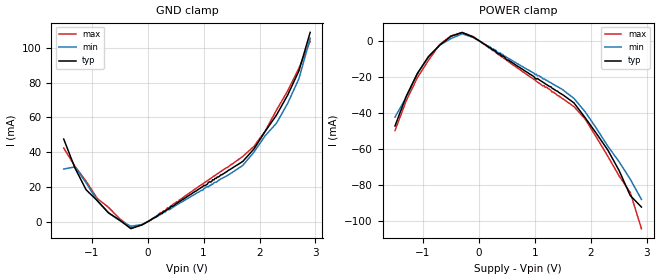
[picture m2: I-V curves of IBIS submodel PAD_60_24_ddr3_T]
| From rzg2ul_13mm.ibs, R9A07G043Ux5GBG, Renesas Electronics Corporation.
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[Submodel]  PAD_60_24_ddr3_T
Submodel_type Dynamic_clamp
[GND Clamp]
| Voltage   I(typ)   I(min)   I(max)
-1.5V     47.49mA    30.28mA    42.32mA
-1.3V     30.91mA    31.46mA    31.89mA
-1.1V     18.34mA    22.35mA    23.25mA
-900mV    12.1mA     12.05mA    13.29mA
-700mV    5.143mA    5.001mA    8.271mA
-300mV    -3.998mA   -2.627mA   -3.451mA
-100mV    -1.794mA   -1.578mA   -1.849mA
1.7V      34.63mA    32.33mA    37.5mA
2.1V      51.84mA    49.38mA    52.03mA
2.505V    72.91mA    68.19mA    75.29mA
2.705V    86.79mA    82.27mA    88.33mA
2.905V    108.8mA    105.5mA    103.7mA
[POWER Clamp]
| Voltage   I(typ)   I(min)   I(max)
-1.5V     -47.33mA   -42.38mA   -49.88mA
-1.3V     -30.9mA    -31.49mA   -33.4mA
-1.1V     -18.19mA   -18.43mA   -20.53mA
-700mV    -2.52mA    -2.471mA   -2.084mA
-300mV    4.482mA    3.775mA    4.566mA
-100mV    1.961mA    1.728mA    2.208mA
1.485V    -29.76mA   -26.91mA   -31.91mA
1.7V      -34.53mA   -32.03mA   -36.58mA
1.9V      -42.75mA   -39.49mA   -43.5mA
2.305V    -60.68mA   -58.51mA   -64.13mA
2.705V    -85.84mA   -76.77mA   -84.17mA
2.905V    -92.22mA   -87.99mA   -104.2mA
